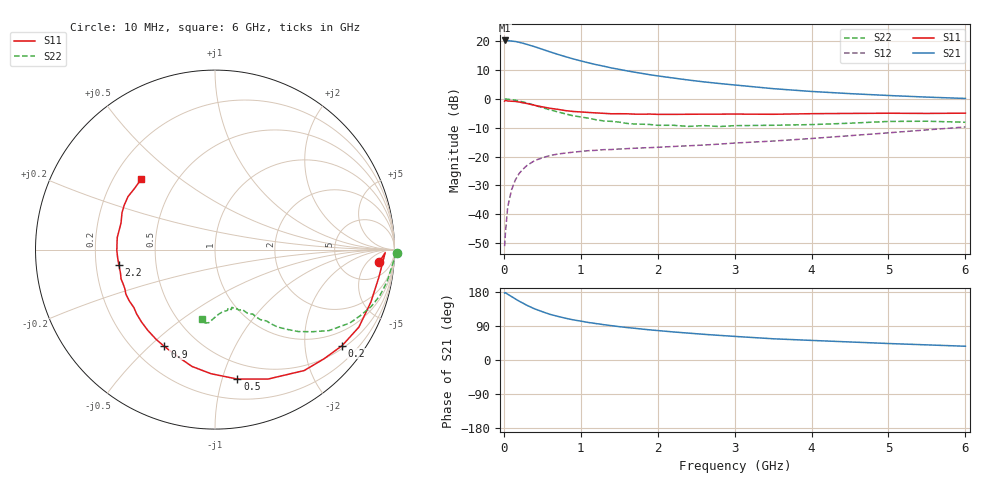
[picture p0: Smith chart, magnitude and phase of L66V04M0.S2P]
!  INFINEON TECHNOLOGIES Small Signal Semiconductors
! BFR380L3 , Si-NPN RF-Transistor in TSLP-3-1
!  Vce=6 V,  Ic=4 mA
! Common Emitter S-Parameters:  07. March 2005
#  GHz  S  MA  R  50
! f  S11  S21  S12  S22
! GHz  Mag  Ang  Mag  Ang  Mag  Ang  Mag  Ang
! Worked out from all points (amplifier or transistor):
!   36 points, 10 MHz to 6 GHz, reference 50 ohm
!   highest |S21| = 20.3 dB at 10 MHz (marker M1)
!   |S21| within 3 dB of that: start of sweep to 493.5 MHz
!   unconditionally stable (mu >= 1): 3.09 GHz to 4.511 GHz
!   at 250 MHz: K = 0.12, MSG = 21.8 dB, |S12| = -24.3 dB
!   at 1.4 GHz: K = 0.65, MSG = 14.2 dB, |S12| = -17.5 dB
!   at 6 GHz: K = 0.91, MSG = 4.9 dB, |S12| = -9.7 dB
!   S11 on the Smith chart (normalised r, x): 10 MHz: 13, -12; 200 MHz: 0.57, -2.89; 500 MHz: 0.36, -1.12; 900 MHz: 0.33, -0.56; 2.2 GHz: 0.30, -0.07; 6 GHz: 0.32, +0.37
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0.01  0.9181 -4.3  10.4 176.9  0.0028 80.7  1.013 -1.1
0.02  0.9485 -1.0  10.32 177.7  0.0046 89.3  1.004 -2.3
0.05  0.9259 -9.6  10.33 173.6  0.0133 85.6  0.9904 -5.3
0.15  0.9106 -28.3  9.978 161.2  0.0395 75.5  0.9533 -15.7
0.2  0.8879 -37.0  9.657 155.1  0.0514 70.9  0.9264 -20.0
0.3  0.8372 -53.6  8.889 144.3  0.0703 62.9  0.856 -28.5
0.4  0.7795 -67.7  8.106 135.0  0.0854 56.3  0.779 -35.4
0.5  0.7321 -80.2  7.311 127.5  0.0956 51.7  0.7102 -40.1
0.6  0.6919 -91.8  6.593 120.5  0.1048 47.8  0.6515 -44.5
0.7  0.6637 -101.1  5.975 115.2  0.111 45.0  0.5988 -47.9
0.8  0.6305 -109.5  5.449 110.3  0.1156 42.8  0.5538 -51.1
0.9  0.6089 -117.6  4.982 106.0  0.1196 41.3  0.5127 -53.2
1.1  0.5854 -129.7  4.253 99.0  0.1271 39.9  0.4656 -57.0
1.3  0.5651 -140.5  3.714 93.2  0.1325 39.1  0.4165 -59.6
1.5  0.5566 -149.0  3.275 88.0  0.1359 39.6  0.3977 -63.0
1.9  0.5484 -162.7  2.64 79.5  0.1435 41.0  0.362 -68.6
2.2  0.5423 -170.7  2.321 74.1  0.1503 42.9  0.351 -70.5
2.8  0.5472 175.9  1.863 65.0  0.1651 47.8  0.3335 -77.4
3.5  0.5442 164.1  1.515 56.0  0.1868 52.1  0.3508 -83.7
4.5  0.5633 153.9  1.242 47.6  0.2315 58.5  0.3811 -90.7
5.5  0.5631 142.7  1.081 39.9  0.2917 60.7  0.4124 -97.6
6  0.5691 136.1  1.024 36.3  0.3277 60.4  0.3955 -100.7
